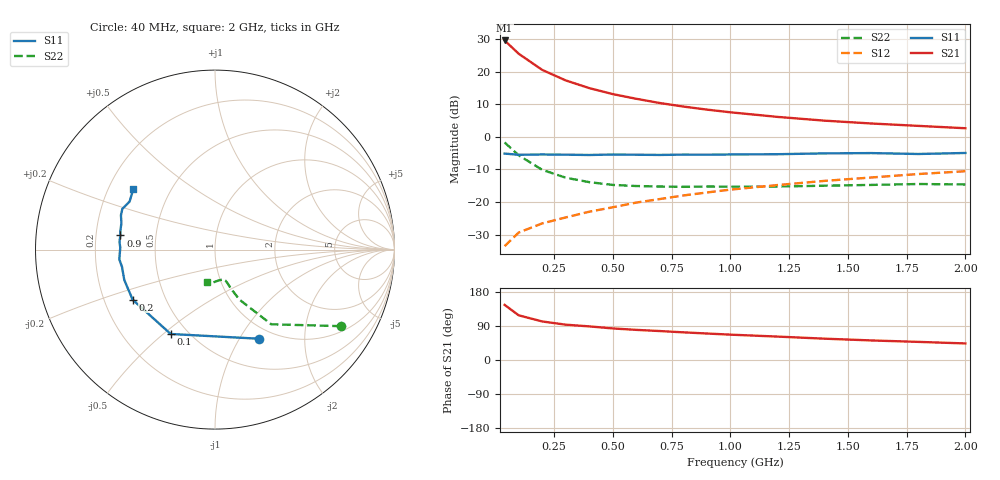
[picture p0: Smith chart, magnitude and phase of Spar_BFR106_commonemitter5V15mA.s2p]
! Filename:  BFR106A.S2P  Version:  2.0
! NXP part #: BFR106  Date: Jun 1990
! Bias condition: Vce=5V, Ic=15mA
#  MHz  S  MA  R  50
! Freq  S11  S21  S12  S22  !GUM [dB]
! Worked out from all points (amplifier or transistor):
!   16 points, 40 MHz to 2 GHz, reference 50 ohm
!   highest |S21| = 29.6 dB at 40 MHz (marker M1)
!   |S21| within 3 dB of that: start of sweep to 84.08 MHz
!   unconditionally stable (mu >= 1): 452.4 MHz to 1.557 GHz; 1.746 GHz to 1.814 GHz
!   at 200 MHz: K = 0.73, MSG = 23.6 dB, |S12| = -26.6 dB
!   at 800 MHz: K = 1.06, MAG = 12.2 dB, |S12| = -18.0 dB
!   at 2 GHz: K = 0.98, MSG = 6.6 dB, |S12| = -10.5 dB
!   S11 on the Smith chart (normalised r, x): 40 MHz: 0.85, -1.22; 100 MHz: 0.40, -0.53; 200 MHz: 0.32, -0.25; 900 MHz: 0.31, +0.07; 2 GHz: 0.30, +0.30
40  0.554 -63.7  30.21 145.5  0.021 66.1  0.821 -31.3
100  0.531 -117.7  18.88 117.9  0.034 53.4  0.521 -53.0
200  0.537 -148.7  10.67 101.7  0.047 55.4  0.312 -63.8
300  0.533 -161.5  7.361 93.2  0.058 58.4  0.236 -67.8
400  0.527 -169.5  5.605 88.7  0.071 62.0  0.202 -69.4
500  0.536 -174.2  4.538 83.3  0.083 64.4  0.183 -71.3
600  0.532 -176.7  3.844 79.5  0.098 66.2  0.176 -73.2
700  0.528 178.7  3.311 76.4  0.111 67.2  0.173 -74.5
800  0.534 175.4  2.922 73.0  0.126 68.2  0.171 -75.3
900  0.533 171.5  2.623 69.9  0.14 69.3  0.173 -76.2
1000  0.537 169.4  2.386 66.9  0.155 68.3  0.172 -78.2
1200  0.542 164.2  2.028 61.8  0.182 68.0  0.173 -83.3
1400  0.558 159.9  1.775 56.3  0.211 67.6  0.178 -88.8
1600  0.564 156.3  1.605 51.6  0.238 67.3  0.183 -92.9
1800  0.546 150.6  1.475 47.8  0.269 66.0  0.189 -98.1
2000  0.566 143.6  1.357 43.7  0.297 65.1  0.186 -104.2
